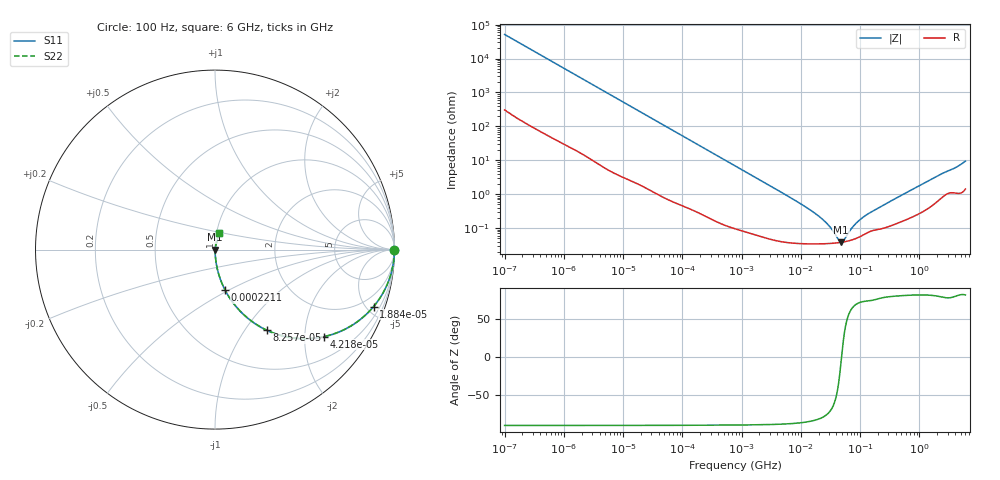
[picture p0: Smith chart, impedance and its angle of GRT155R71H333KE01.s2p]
!Murata Part Number: GRT155R71H333KE01
!These Parameters are Measured in Series Mode Connection
!Data Generated on Jun 19, 2026
!  o--ll--o
!Port1  Port2
!  o------o
!Operation Temp=25[degC], DC Bias Voltage=0[V]
!Freq. Start=100[Hz] Stop=6[GHz] 401[Steps]
# Hz S RI R 50
!Freq.(Hz) S11(Real) S11(Imag) S21(Real) S21(Imag) S12(Real) S12(Imag) S22(Real) S22(Imag)
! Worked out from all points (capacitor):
!   401 points, 100 Hz to 6 GHz, reference 50 ohm
!   read as one part in series: C = 30.9 nF near 109 Hz
!   lowest |Z| = 38.4 mohm at 47.65 MHz (marker M1)
!   series resonance near 48.73 MHz, so ESL is about 340 pH
!   S11 on the Smith chart (normalised r, x): 100 Hz: open; 18.84 kHz: 1.04, -5.55; 42.18 kHz: 1.02, -2.49; 82.57 kHz: 1.01, -1.27; 221.1 kHz: 1.00, -0.48; 6 GHz: 1.03, +0.19
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100  1 -0.00195  1.54e-05 0.00195  1.54e-05 0.00195  1 -0.00195
2008  0.9983 -0.0386  0.00173 0.0386  0.00173 0.0386  0.9983 -0.0386
6728  0.9829 -0.1268  0.0171 0.1268  0.0171 0.1268  0.9829 -0.1268
18841  0.8835 -0.3175  0.1165 0.3175  0.1165 0.3175  0.8835 -0.3175
26957  0.789 -0.4045  0.211 0.4045  0.211 0.4045  0.789 -0.4045
40335  0.6278 -0.4798  0.3722 0.4798  0.3722 0.4798  0.6278 -0.4798
42182  0.6069 -0.4848  0.3931 0.4848  0.3931 0.4848  0.6069 -0.4848
57709  0.4537 -0.4941  0.5463 0.4941  0.5463 0.4941  0.4537 -0.4941
82567  0.2905 -0.4499  0.7095 0.4499  0.7095 0.4499  0.2905 -0.4499
129199  0.1452 -0.3477  0.8548 0.3477  0.8548 0.3477  0.1452 -0.3477
221108  0.0563 -0.2254  0.9437 0.2254  0.9437 0.2254  0.0563 -0.2254
774597  0.00565 -0.0683  0.9943 0.0683  0.9943 0.0683  0.00565 -0.0683
6075234  0.00045 -0.00874  0.9996 0.00874  0.9996 0.00874  0.00045 -0.00874
1.555665e7  0.000352 -0.00312  0.9996 0.00312  0.9996 0.00312  0.000352 -0.00312
2.784235e7  0.000351 -0.00131  0.9996 0.00131  0.9996 0.00131  0.000351 -0.00131
4.35672e7  0.000372 -0.000248  0.9996 0.000248  0.9996 0.000248  0.000372 -0.000248
4.764863e7  0.00038 -4.91e-05  0.9996 4.91e-05  0.9996 4.91e-05  0.00038 -4.91e-05
5.211241e7  0.00039 0.000149  0.9996 -0.000149  0.9996 -0.000149  0.00039 0.000149
7.455971e7  0.000455 0.000961  0.9995 -0.000961  0.9995 -0.000961  0.000455 0.000961
1.020051e8  0.000573 0.00174  0.9994 -0.00174  0.9994 -0.00174  0.000573 0.00174
3.124326e8  0.00116 0.00585  0.9988 -0.00585  0.9988 -0.00585  0.00116 0.00585
6e9  0.0223 0.0901  0.9777 -0.0901  0.9777 -0.0901  0.0223 0.0901
